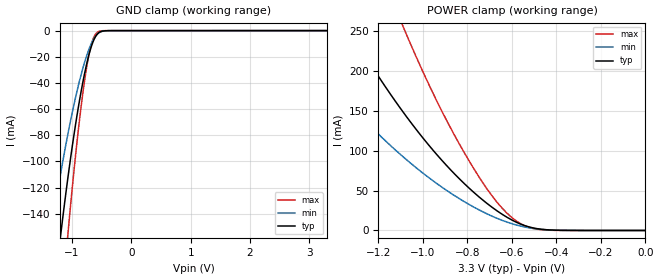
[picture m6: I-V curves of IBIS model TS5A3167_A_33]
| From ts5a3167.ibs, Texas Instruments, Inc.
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[Model]   TS5A3167_A_33
Model_type  Terminator
| variable   typ   min   max
C_comp   18.61pF   16.80pF   20.11pF
| C_tri-state   18.61pF   16.80pF   20.11pF
[Temperature Range]   40   100   -40
| Ambient temperature   25   85   -40
[Voltage range]   3.3   3   3.6
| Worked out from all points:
|   GND clamp passes 1 mA (typ) near -0.53 V on its own axis
|   POWER clamp passes 1 mA (typ) near -0.45 V on its own axis
[GND Clamp]
| TS5A3167_A_33
|   Voltage   I(typ)   I(min)   I(max)
-3.3V     -1.34A     -980.7mA   -1.797A
-1.365V   -226.5mA   -157.8mA   -322.3mA
-1.335V   -213.8mA   -148.9mA   -303.9mA
-1.185V   -153.8mA   -107.5mA   -216.7mA
-1.07V    -112.6mA   -79.14mA   -155.9mA
-900mV    -60.43mA   -43.27mA   -78.61mA
-775mV    -29.99mA   -22.28mA   -34.17mA
-725mV    -20.23mA   -15.51mA   -20.75mA
-670mV    -11.57mA   -9.396mA   -9.881mA
-620mV    -5.935mA   -5.234mA   -3.907mA
-555mV    -1.857mA   -1.921mA   -769.7uA
3.3V      962.9pA    34.74uA    63.63pA
[POWER Clamp]
| TS5A3167_A_33
|   Voltage   I(typ)   I(min)   I(max)
-3.3V     1.641A     1.143A     2.481A
-1.62V    401.2mA    256.2mA    676mA
-1.59V    384.5mA    245.2mA    649.1mA
-1.33V    251.2mA    158mA      430.5mA
-1.09V    148.6mA    92.45mA    255.9mA
-1.07V    141mA      87.67mA    242.7mA
-950mV    98.99mA    61.23mA    169.1mA
-815mV    58.91mA    36.22mA    97.8mA
-700mV    31.27mA    19.23mA    47.28mA
-600mV    13.07mA    8.467mA    16.08mA
-465mV    1.423mA    1.287mA    867.9uA
-48.03fV  962.9pA    7.155nA    83.57pA
